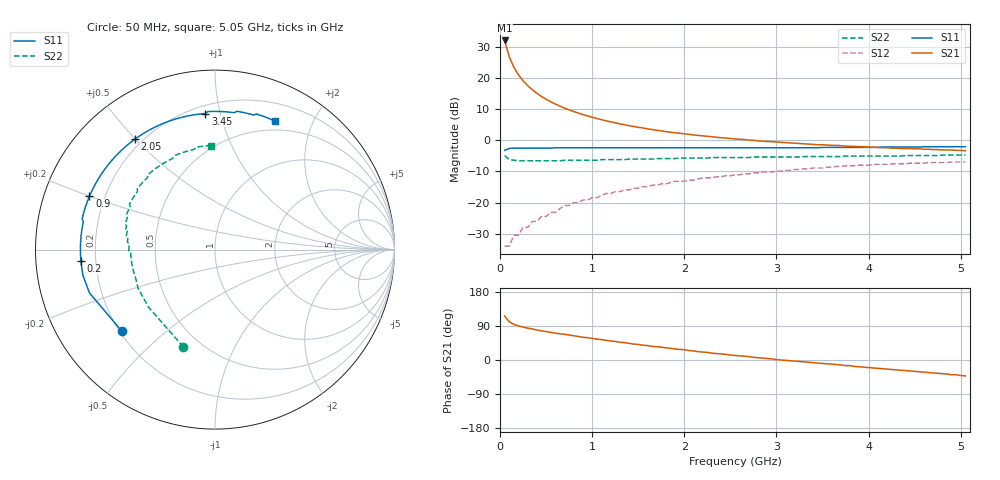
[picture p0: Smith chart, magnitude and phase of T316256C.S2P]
!AT-31625
!S-PARAMETERS at Vce=6.0 V  Ic=150 mA.  LAST UPDATED 08-05-96
# ghz s ma r 50
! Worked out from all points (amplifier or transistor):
!   101 points, 50 MHz to 5.05 GHz, reference 50 ohm
!   highest |S21| = 32.1 dB at 50 MHz (marker M1)
!   |S21| within 3 dB of that: start of sweep to 78.72 MHz
!   unconditionally stable (mu >= 1): 397.6 MHz to 407.2 MHz; 465.5 MHz to 1.859 GHz
!   at 850 MHz: K = 1.03, MAG = 13.3 dB, |S12| = -20.0 dB
!   at 2.55 GHz: K = 0.97, MSG = 5.7 dB, |S12| = -11.1 dB
!   at 5.05 GHz: K = 0.94, MSG = 1.8 dB, |S12| = -6.9 dB
!   S11 on the Smith chart (normalised r, x): 50 MHz: 0.21, -0.36; 200 MHz: 0.14, -0.04; 900 MHz: 0.14, +0.20; 2.05 GHz: 0.17, +0.50; 3.45 GHz: 0.25, +0.90; 5.05 GHz: 0.39, +1.50
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0.05  0.69 -139.0  40.12 116.0  0.02 42.0  0.57 -108.0
0.1  0.74 -161.0  21.99 101.0  0.02 42.0  0.49 -139.0
0.15  0.75 -169.0  14.91 94.0  0.03 47.0  0.48 -153.0
0.2  0.75 -175.0  11.26 90.0  0.03 52.0  0.47 -160.0
0.25  0.75 -178.0  9.05 87.0  0.04 55.0  0.47 -164.0
0.3  0.75 179.0  7.56 84.0  0.04 58.0  0.47 -168.0
0.35  0.75 176.0  6.5 82.0  0.05 60.0  0.47 -170.0
0.4  0.75 174.0  5.69 79.0  0.05 61.0  0.47 -172.0
0.45  0.75 172.0  5.07 77.0  0.06 62.0  0.47 -173.0
0.55  0.75 168.0  4.17 73.0  0.07 63.0  0.47 -176.0
0.65  0.76 165.0  3.54 69.0  0.08 63.0  0.47 -178.0
0.75  0.76 162.0  3.08 66.0  0.09 63.0  0.48 -180.0
0.9  0.76 157.0  2.59 60.0  0.11 62.0  0.48 178.0
1.05  0.76 153.0  2.24 55.0  0.12 60.0  0.48 176.0
1.3  0.76 146.0  1.84 47.0  0.15 57.0  0.49 173.0
1.75  0.76 134.0  1.42 34.0  0.2 50.0  0.51 167.0
2.05  0.76 126.0  1.25 25.0  0.23 45.0  0.52 163.0
2.55  0.76 114.0  1.05 12.0  0.28 36.0  0.53 155.0
3.4  0.76 95.0  0.86 -7.0  0.36 21.0  0.55 140.0
3.45  0.76 94.0  0.85 -8.0  0.36 20.0  0.55 139.0
4.25  0.78 79.0  0.75 -25.0  0.42 3.0  0.56 118.0
5.05  0.79 65.0  0.68 -42.0  0.45 -14.0  0.58 92.0
